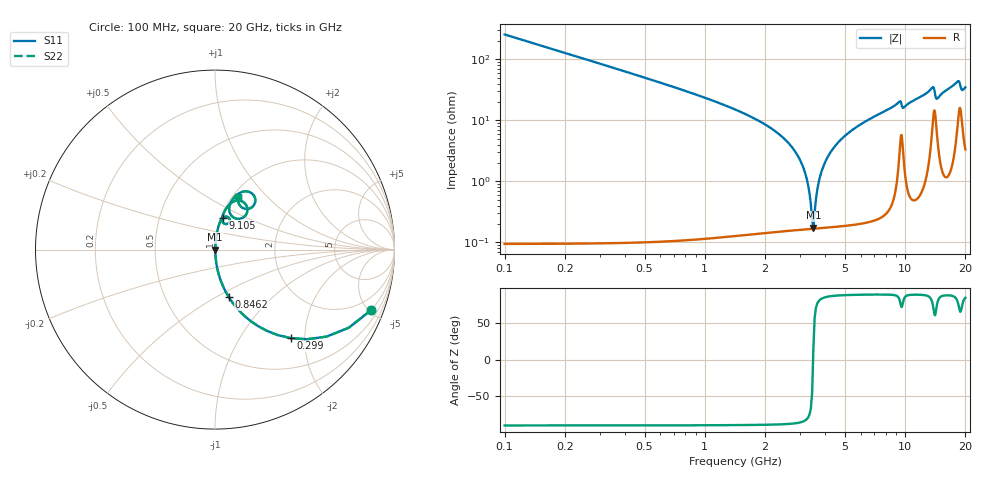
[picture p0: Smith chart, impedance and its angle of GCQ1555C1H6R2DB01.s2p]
!Murata Part Number: GCQ1555C1H6R2DB01
!These Parameters are Measured in Series Mode Connection
!Data Generated on Jan 08, 2026
!  o--ll--o
!Port1  Port2
!  o------o
!Operation Temp=25[degC], DC Bias Voltage=0[V]
!Freq. Start=100[MHz] Stop=20[GHz] 401[Steps]
# Hz S RI R 50
!Freq.(Hz) S11(Real) S11(Imag) S21(Real) S21(Imag) S12(Real) S12(Imag) S22(Real) S22(Imag)
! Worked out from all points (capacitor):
!   401 points, 100 MHz to 20 GHz, reference 50 ohm
!   read as one part in series: C = 6.2 pF near 199.5 MHz
!   lowest |Z| = 173 mohm at 3.483 GHz (marker M1)
!   series resonance near 3.472 GHz, so ESL is about 340 pH
!   S11 on the Smith chart (normalised r, x): 100 MHz: 1.00, -5.13; 299 MHz: 1.00, -1.70; 846.2 MHz: 1.00, -0.57; 9.105 GHz: 1.02, +0.37; 20 GHz: 1.07, +0.69
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1e8  0.868 -0.3384  0.132 0.3384  0.132 0.3384  0.868 -0.3384
2.99e8  0.4207 -0.4931  0.5793 0.4931  0.5793 0.4931  0.4207 -0.4931
4.98e8  0.2035 -0.4016  0.7965 0.4016  0.7965 0.4016  0.2035 -0.4016
8.4625e8  0.0761 -0.2632  0.9239 0.2632  0.9239 0.2632  0.0761 -0.2632
2.289e9  0.00546 -0.0629  0.9945 0.0629  0.9945 0.0629  0.00546 -0.0629
2.83625e9  0.00248 -0.03  0.9975 0.03  0.9975 0.03  0.00248 -0.03
3.1845e9  0.00179 -0.0128  0.9982 0.0128  0.9982 0.0128  0.00179 -0.0128
3.43325e9  0.00166 -0.00167  0.9983 0.00167  0.9983 0.00167  0.00166 -0.00167
3.483e9  0.00167 0.000455  0.9983 -0.000455  0.9983 -0.000455  0.00167 0.000455
3.83125e9  0.00192 0.0145  0.9981 -0.0145  0.9981 -0.0145  0.00192 0.0145
4.32875e9  0.00285 0.0328  0.9971 -0.0328  0.9971 -0.0328  0.00285 0.0328
5.274e9  0.00597 0.0637  0.994 -0.0637  0.994 -0.0637  0.00597 0.0637
6.7665e9  0.0137 0.1066  0.9863 -0.1066  0.9863 -0.1066  0.0137 0.1066
9.10475e9  0.0425 0.1766  0.9575 -0.1766  0.9575 -0.1766  0.0425 0.1766
1.005e10  0.039 0.1641  0.961 -0.1641  0.961 -0.1641  0.039 0.1641
1.338325e10  0.1161 0.272  0.8839 -0.272  0.8839 -0.272  0.1161 0.272
1.3831e10  0.1756 0.2444  0.8244 -0.2444  0.8244 -0.2444  0.1756 0.2444
1.437825e10  0.0993 0.1819  0.9007 -0.1819  0.9007 -0.1819  0.0993 0.1819
1.67165e10  0.1134 0.2976  0.8866 -0.2976  0.8866 -0.2976  0.1134 0.2976
1.8607e10  0.2246 0.2762  0.7754 -0.2762  0.7754 -0.2762  0.2246 0.2762
1.915425e10  0.1581 0.2304  0.8419 -0.2304  0.8419 -0.2304  0.1581 0.2304
2e10  0.1306 0.2922  0.8694 -0.2922  0.8694 -0.2922  0.1306 0.2922
